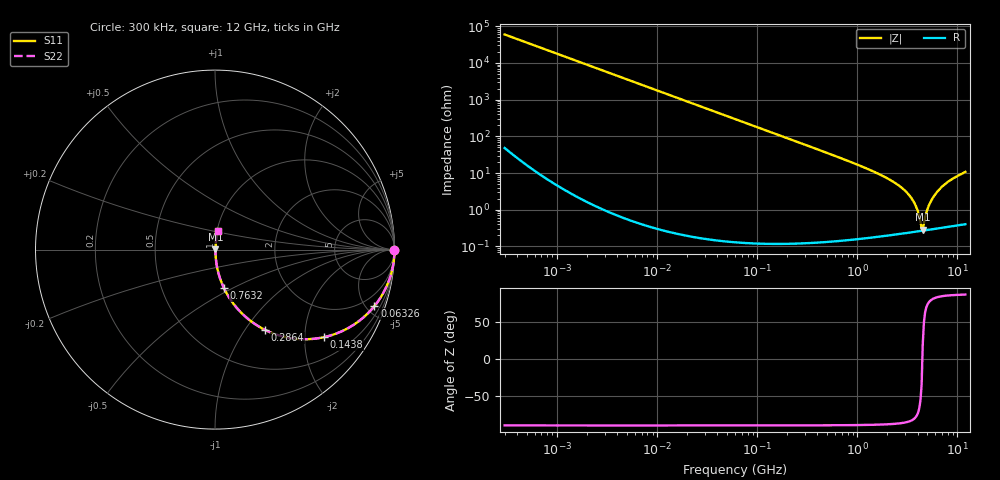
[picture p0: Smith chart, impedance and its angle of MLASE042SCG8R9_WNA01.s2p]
! MLASE042SCG8R9_WNA01  S-PARAMETER MODEL  ( General Type )
! Model Generated by TAIYO YUDEN Corporation (http://www.ty-top.com)
! Version 1.0
! TAIYO YUDEN Control No. 130801
! Copyright(c) 2013 TAIYO YUDEN CO.,LTD. All Rights Reserved.
! Product Description (link to TY-COMPAS)
! https://ds.yuden.co.jp/TYCOMPAS/or/detail?pn=MLASE042SCG8R9BWNA01&u=M
! Products Name : Multilayer Ceramic Capacitors
! Characteristics :
!  Capacitance : 8.9 pF , Rated Voltage : 16V , TCC : CG / C0G
!  Case Size : 0.4 x 0.2 / 0.016 x 0.008 [mm/inch] , Thickness : 0.2 / 0.008 [mm/inch]
!  (Conditions: Temperature = 25 degC , DC Bias Current/Voltage = 0A / 0V)
! External Node Assignments :
!  1  o---| |---o  2
! GND o---------o GND
! Frequency Range : 0.3MHz  -  12000MHz  [ 401 STEP ]
# MHz S RI R 50
! Freq[MHz].  S11 Real  S11 Imag  S21 Real  S21 Imag  S12 Real  S12 Imag  S22 Real  S22 Imag
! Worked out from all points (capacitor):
!   401 points, 300 kHz to 12 GHz, reference 50 ohm
!   read as one part in series: C = 8.9 pF near 316.3 kHz
!   lowest |Z| = 289 mohm at 4.503 GHz (marker M1)
!   series resonance near 4.461 GHz, so ESL is about 140 pH
!   S11 on the Smith chart (normalised r, x): 300 kHz: open; 63.26 MHz: 1.00, -5.65; 143.8 MHz: 1.00, -2.48; 286.4 MHz: 1.00, -1.24; 763.2 MHz: 1.00, -0.45; 12 GHz: 1.01, +0.22
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0.3  1 -0.00168  4.17e-06 0.00168  4.17e-06 0.00168  1 -0.00168
1.769972  0.9999 -0.0099  9.99e-05 0.0099  9.99e-05 0.0099  0.9999 -0.0099
10.44266  0.9966 -0.0582  0.00341 0.0582  0.00341 0.0582  0.9966 -0.0582
26.39317  0.9786 -0.1445  0.0214 0.1445  0.0214 0.1445  0.9786 -0.1445
60  0.8986 -0.3017  0.1014 0.3017  0.1014 0.3017  0.8986 -0.3017
63.26471  0.8885 -0.3145  0.1115 0.3145  0.1115 0.3145  0.8885 -0.3145
143.8206  0.6064 -0.4881  0.3936 0.4881  0.3936 0.4881  0.6064 -0.4881
286.3882  0.2791 -0.4476  0.7209 0.4476  0.7209 0.4476  0.2791 -0.4476
353.9943  0.2017 -0.4  0.7983 0.4  0.7983 0.4  0.2017 -0.4
763.2128  0.0504 -0.2156  0.9496 0.2156  0.9496 0.2156  0.0504 -0.2156
2088.533  0.00645 -0.0664  0.9935 0.0664  0.9935 0.0664  0.00645 -0.0664
2795.104  0.00375 -0.0389  0.9962 0.0389  0.9962 0.0389  0.00375 -0.0389
3364.605  0.00293 -0.0231  0.9971 0.0231  0.9971 0.0231  0.00293 -0.0231
3841.137  0.00268 -0.0123  0.9973 0.0123  0.9973 0.0123  0.00268 -0.0123
4270.516  0.00265 -0.00386  0.9973 0.00386  0.9973 0.00386  0.00265 -0.00386
4502.883  0.00269 0.00103  0.9973 -0.00103  0.9973 -0.00103  0.00269 0.00103
4623.766  0.00273 0.00327  0.9973 -0.00327  0.9973 -0.00327  0.00273 0.00327
5006.236  0.0029 0.00972  0.9971 -0.00972  0.9971 -0.00972  0.0029 0.00972
5278.635  0.00308 0.0143  0.9969 -0.0143  0.9969 -0.0143  0.00308 0.0143
6354.153  0.00412 0.0319  0.9959 -0.0319  0.9959 -0.0319  0.00412 0.0319
8281.503  0.00715 0.0606  0.9929 -0.0606  0.9929 -0.0606  0.00715 0.0606
12000  0.0155 0.1062  0.9845 -0.1062  0.9845 -0.1062  0.0155 0.1062
